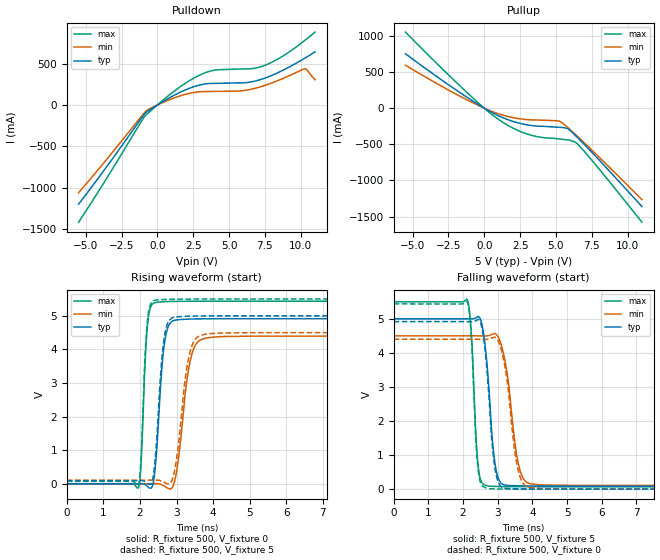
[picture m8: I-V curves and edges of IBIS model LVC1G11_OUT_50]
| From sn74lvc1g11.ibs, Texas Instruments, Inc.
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[Model]   LVC1G11_OUT_50
Model_type  Output
Vref =   0
Rref =   500
Cref =   50p
Vmeas =   2.5
| variable   typ   min   max
C_comp   7.88pF   5.92pF   9.56pF
| C_pullup   8.30pF   5.92pF   9.56pF
| C_pulldown   7.45pF   6.07pF   9.35pF
[Temperature Range]   40   100   -40
| Ambient temperature   25   85   -40
[Voltage range]   5   4.5   5.5
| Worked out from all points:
|   slope of the pulldown table from 0 to 0.75 V, typ, clamps not added: 9.58 ohm
|   slope of the pullup table from 0 to 0.75 V, typ, clamps not added: 9.16 ohm
|   rising waveform, R_fixture 500, V_fixture 0: 20-80 % time 186ps typ, 279ps min, 127ps max; typ from 0 V to 4.91 V
|   falling waveform, R_fixture 500, V_fixture 5: 20-80 % time 224ps typ, 315ps min, 147ps max; typ from 5 V to 0.09 V
|   rising waveform, R_fixture 500, V_fixture 5: 20-80 % time 184ps typ, 276ps min, 125ps max; typ from 0.09 V to 5 V
|   falling waveform, R_fixture 500, V_fixture 0: 20-80 % time 221ps typ, 307ps min, 146ps max; typ from 4.92 V to 0 V
[Pulldown]
| LVC1G11_OUT_50
|   Voltage   I(typ)   I(min)   I(max)
-5.5V     -1.198A    -1.059A    -1.415A
-940mV    -118.4mA   -100.1mA   -148.6mA
-645mV    -71.01mA   -53.56mA   -98.24mA
800mV     83.29mA    61.2mA     116.9mA
2.295V    206.2mA    143.4mA    300.5mA
3.555V    259mA      163mA      402.9mA
5.915V    268.2mA    172.5mA    435.1mA
6.785V    288mA      200.6mA    444mA
7.565V    329.2mA    240.8mA    484mA
8.805V    423.4mA    324.2mA    597mA
10.28V    565mA      437.4mA    779.4mA
11V       641.2mA    305.2mA    880.8mA
[Pullup]
| LVC1G11_OUT_50
|   Voltage   I(typ)   I(min)   I(max)
-5.5V     752.7mA    594.4mA    1.054A
-1.36V    171.1mA    130.8mA    245.1mA
125mV     -14.77mA   -11.04mA   -21.53mA
1.015V    -107mA     -78.37mA   -158.2mA
2.025V    -184.2mA   -131mA     -278mA
3.04V     -232.4mA   -158.5mA   -360.7mA
3.945V    -250.5mA   -165.3mA   -402.5mA
5.3V      -265.9mA   -185.4mA   -427.7mA
5.83V     -285.1mA   -268.2mA   -440mA
6.53V     -411.2mA   -395.2mA   -500.3mA
8.1V      -736mA     -695.6mA   -863mA
11V       -1.361A    -1.267A    -1.578A
[Ramp]
| LVC1G11_OUT_50
| variable   typ   min   max
dV/dt_r   3.03/1.95E-10   2.73/2.92E-10   3.33/1.32E-10
dV/dt_f   2.99/2.32E-10   2.68/3.31E-10   3.31/1.52E-10
R_load = 500
[Rising Waveform]
| LVC1G11_OUT_50
R_fixture =   500
C_fixture =   0
L_fixture =   0
V_fixture =   0
V_fixture_min = 0
V_fixture_max = 0
|   Time   V(typ)   V(min)   V(max)
0s        181.8pV    4.248nV    2.382nV
1.96ns    2.035mV    -57.65uV   -115.3mV
2.03ns    5.25mV     -153.3uV   597mV
2.205ns   -77.7mV    87.22uV    4.71V
2.43ns    630.6mV    4.502mV    5.397V
2.67ns    4.178V     -71.6mV    5.421V
2.98ns    4.877V     238.1mV    5.431V
3.38ns    4.905V     3.689V     5.434V
3.81ns    4.912V     4.34V      5.435V
24.99ns   4.914V     4.397V     5.435V
[Falling Waveform]
| LVC1G11_OUT_50
R_fixture =   500
C_fixture =   0
L_fixture =   0
V_fixture =   5
V_fixture_min = 4.5
V_fixture_max = 5.5
|   Time   V(typ)   V(min)   V(max)
0s        5V         4.5V       5.5V
2.125ns   4.999V     4.5V       5.56V
2.245ns   4.997V     4.5V       4.491V
2.435ns   5.071V     4.499V     697.4mV
2.69ns    3.686V     4.499V     100mV
2.865ns   1.249V     4.552V     82.11mV
3.01ns    338.1mV    4.475V     78.34mV
3.605ns   99.53mV    703.5mV    72.75mV
3.96ns    93.13mV    155.8mV    71.91mV
24.99ns   89.63mV    107.6mV    71.34mV
[Rising Waveform]
| LVC1G11_OUT_50
R_fixture =   500
C_fixture =   0
L_fixture =   0
V_fixture =   5
V_fixture_min = 4.5
V_fixture_max = 5.5
|   Time   V(typ)   V(min)   V(max)
0s        89.62mV    107.6mV    71.33mV
1.96ns    91.66mV    107.5mV    -23.34mV
2.025ns   94.57mV    107.5mV    681.9mV
2.195ns   26.64mV    107.6mV    4.753V
2.42ns    784.2mV    112.3mV    5.467V
2.655ns   4.286V     51.1mV     5.486V
2.97ns    4.967V     519.9mV    5.496V
3.34ns    4.991V     3.791V     5.499V
3.755ns   4.998V     4.447V     5.5V
24.99ns   5V         4.5V       5.5V
[Falling Waveform]
| LVC1G11_OUT_50
R_fixture =   500
C_fixture =   0
L_fixture =   0
V_fixture =   0
V_fixture_min = 0
V_fixture_max = 0
|   Time   V(typ)   V(min)   V(max)
0s        4.917V     4.401V     5.437V
2.125ns   4.917V     4.401V     5.492V
2.24ns    4.914V     4.401V     4.461V
2.43ns    4.986V     4.4V       628.4mV
2.685ns   3.561V     4.399V     27.32mV
2.855ns   1.166V     4.447V     10.36mV
3.005ns   231.9mV    4.368V     6.565mV
3.575ns   9.693mV    631.5mV    1.446mV
3.95ns    3.301mV    42.57mV    568.5uV
24.99ns   10.7uV     14.29uV    11.54uV
